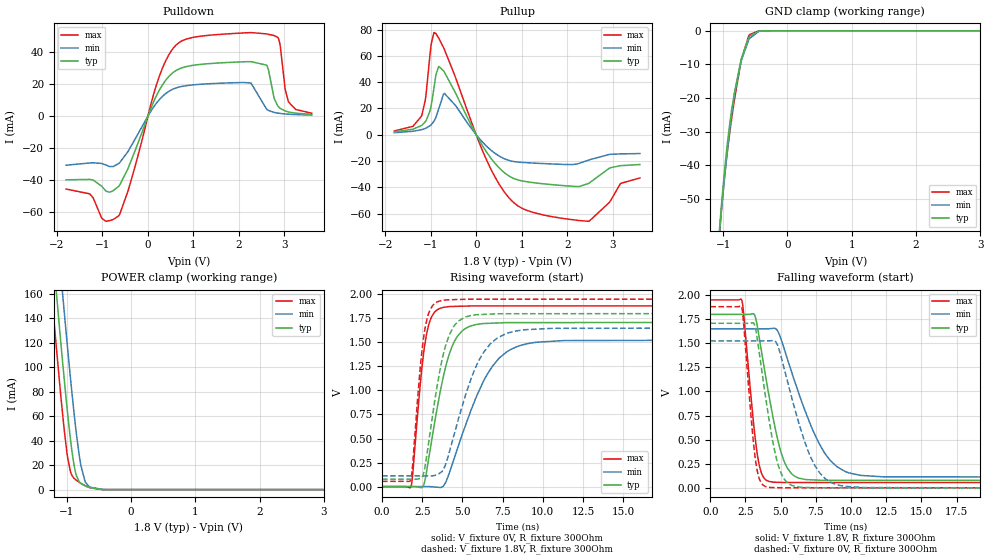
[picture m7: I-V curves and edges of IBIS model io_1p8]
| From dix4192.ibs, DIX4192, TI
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|   io_1p8 Model
[Model]   io_1p8
Model_type   3-state
Polarity   Non-Inverting
Vmeas = 0.9
Vref = 0
Cref = 2pF
Rref = 100000
|   typ   min   max
C_comp   31.7424pF   25.9198pF   37.639pF
|C_comp_pullup   32.4818pF   26.524pF   38.1625pF
|C_comp_pulldown   32.184pF   26.3999pF   37.9873pF
| Where nom  PVT is Nominal Process, 1.8V, 27C
|   Fast PVT is Strong Process,  1.95V, -40C
|   Slow PVT is Weak Process,   1.65V, 105C
[Voltage Range]   1.8   1.65   1.95
[Temperature Range]   27   105   -40
[Pullup Reference]   1.8   1.65   1.95
[Pulldown Reference]   0   0   0
[Power Clamp Reference]   1.8   1.65   1.95
[GND Clamp Reference]   0   0   0
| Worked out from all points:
|   slope of the pulldown table from 0 to 0.27 V, typ, clamps not added: 15.7 ohm
|   slope of the pullup table from 0 to 0.27 V, typ, clamps not added: 17.7 ohm
|   GND clamp passes 1 mA (typ) near -0.53 V on its own axis
|   POWER clamp passes 1 mA (typ) near -0.56 V on its own axis
|   falling waveform, V_fixture 1.8V, R_fixture 300Ohm: 20-80 % time 1.33ns typ, 2.43ns min, 748ps max; typ from 1.8 V to 0.077 V
|   rising waveform, V_fixture 0V, R_fixture 300Ohm: 20-80 % time 1.21ns typ, 2.24ns min, 658ps max; typ from 0 V to 1.71 V
|   rising waveform, V_fixture 1.8V, R_fixture 300Ohm: 20-80 % time 1.07ns typ, 1.84ns min, 606ps max; typ from 0.077 V to 1.8 V
|   falling waveform, V_fixture 0V, R_fixture 300Ohm: 20-80 % time 1.12ns typ, 1.89ns min, 659ps max; typ from 1.71 V to 0 V
[Pulldown]
|   Voltage   I(typ)   I(min)   I(max)
-1.8V     -39.9mA    -30.73mA   -45.65mA
-1.282V   -39.6mA    -29.34mA   -48.64mA
-925.2mV  -46.91mA   -30.57mA   -65.81mA
-644.4mV  -43.96mA   -29.72mA   -62.43mA
273.6mV   17.4mA     10.99mA    26.7mA
538.2mV   26.88mA    16.71mA    41.79mA
840.6mV   30.92mA    18.98mA    48.11mA
2.266V    34.03mA    20.63mA    52.22mA
2.612V    31.83mA    4.169mA    51.37mA
2.855V    6.344mA    1.84mA     49.25mA
3.087V    2.59mA     1.171mA    9.115mA
3.6V      1.075mA    640.9uA    1.804mA
[GND Clamp]
|   Voltage   I(typ)   I(min)   I(max)
-1.8V     -269.5mA   -244.4mA   -304.6mA
-1.076V   -63.64mA   -64.2mA    -65.25mA
-1.028V   -52.24mA   -53.82mA   -53.43mA
-979.2mV  -41.88mA   -44.02mA   -43.51mA
-930.6mV  -32.88mA   -35mA      -35.28mA
-892.8mV  -26.95mA   -28.67mA   -29.64mA
-828mV    -18.71mA   -19.53mA   -20.92mA
-714.6mV  -8.146mA   -8.682mA   -8.428mA
-590.4mV  -1.599mA   -2.281mA   -1.13mA
-444.6mV  -52.32uA   -160.2uA   -14.34uA
-358.2mV  -3.674uA   -21.45uA   -306.9nA
3.6V      0A         0A         0A
[Pullup]
|   Voltage   I(typ)   I(min)   I(max)
-1.8V     2.198mA    1.55mA     2.867mA
-1.201V   7.084mA    3.863mA    14.25mA
-1.114V   10.13mA    4.875mA    27.64mA
-1.017V   18.04mA    6.818mA    60.52mA
-925.2mV  36.38mA    10.47mA    77.67mA
-822.6mV  51.95mA    19.8mA     73.34mA
-698.4mV  47.53mA    31.43mA    64.82mA
235.8mV   -13.6mA    -8.983mA   -19.78mA
916.2mV   -34.35mA   -20.76mA   -54.04mA
2.482V    -36.78mA   -19.12mA   -65.77mA
3.173V    -23.5mA    -14.57mA   -37mA
3.6V      -22.66mA   -14.3mA    -32.84mA
[POWER Clamp]
|   Voltage   I(typ)   I(min)   I(max)
-1.8V     564.8mA    620.9mA    520.8mA
-1.233V   204.8mA    261.9mA    159.6mA
-1.168V   165.5mA    222.3mA    120.5mA
-1.087V   117.7mA    173.8mA    74.13mA
-1.039V   90.27mA    145.4mA    48.83mA
-984.6mV  61.6mA     114.7mA    25.82mA
-941.4mV  40.98mA    91.12mA    14.65mA
-887.4mV  20.49mA    63.43mA    9.326mA
-806.4mV  6.463mA    28.45mA    6.043mA
-714.6mV  3.048mA    6.727mA    3.292mA
-412.2mV  29.86uA    75.19uA    8.803uA
3.6V      0A         0A         0A
[Ramp]
R_load = 300
|   typ   min   max
dV/dt_r   1.02457/1.21031e-09   0.91469/2.23132e-09   1.12794/6.56815e-10
dV/dt_f   1.03368/1.33169e-09   0.923165/2.42115e-09   1.13713/7.46052e-10
[Falling Waveform]
V_fixture = 1.8V
V_fixture_min = 1.65V
V_fixture_max = 1.95V
R_fixture = 300Ohm
C_fixture = 0F
|   Time   V(typ)   V(min)   V(max)
0s        1.8V       1.65V      1.95V
2.24ns    1.8V       1.65V      1.945V
3.307ns   1.703V     1.65V      379.8mV
3.63ns    1.422V     1.65V      155.7mV
4.061ns   1.045V     1.65V      72.4mV
4.946ns   409.7mV    1.575V     57.01mV
5.735ns   152.8mV    1.22V      55.53mV
7.707ns   79.69mV    467mV      55.45mV
9.593ns   78.43mV    169.1mV    55.38mV
25ns      77.2mV     111.4mV    54.79mV
[Rising Waveform]
V_fixture = 0V
V_fixture_min = 0V
V_fixture_max = 0V
R_fixture = 300Ohm
C_fixture = 0F
|   Time   V(typ)   V(min)   V(max)
0s        -681.6nV   4.501uV    -1.632uV
1.797ns   166.2uV    70.36uV    -3.309mV
2.703ns   94.49mV    103.6uV    1.523V
3.029ns   419.9mV    -952.5uV   1.745V
3.566ns   940.3mV    -8.388mV   1.851V
4.193ns   1.383V     147.5mV    1.873V
4.977ns   1.619V     538.1mV    1.877V
6.527ns   1.698V     1.163V     1.879V
8.405ns   1.706V     1.457V     1.879V
25ns      1.708V     1.524V     1.88V
[Rising Waveform]
V_fixture = 1.8V
V_fixture_min = 1.65V
V_fixture_max = 1.95V
R_fixture = 300Ohm
C_fixture = 0F
|   Time   V(typ)   V(min)   V(max)
0s        77.2mV     111.4mV    54.79mV
1.784ns   76.81mV    111.1mV    70.85mV
2.6ns     147.9mV    110.9mV    1.567V
2.923ns   485.6mV    110.9mV    1.813V
3.444ns   1.064V     123.5mV    1.922V
3.982ns   1.482V     246.4mV    1.941V
4.751ns   1.721V     702.9mV    1.946V
6.105ns   1.79V      1.336V     1.949V
7.707ns   1.798V     1.591V     1.949V
25ns      1.8V       1.65V      1.95V
[Falling Waveform]
|Gnd
V_fixture = 0V
V_fixture_min = 0V
V_fixture_max = 0V
R_fixture = 300Ohm
C_fixture = 0F
|   Time   V(typ)   V(min)   V(max)
0s        1.708V     1.524V     1.88V
2.23ns    1.707V     1.524V     1.874V
3.211ns   1.655V     1.524V     287.1mV
3.471ns   1.409V     1.524V     99.7mV
3.856ns   1.011V     1.524V     18.19mV
4.61ns    357.2mV    1.522V     2.764mV
5.261ns   89.47mV    1.23V      760.3uV
7.054ns   3.3mV      344.1mV    691.1uV
8.688ns   1.008mV    48.81mV    628uV
25ns      -658.1nV   4.349uV    -1.601uV
